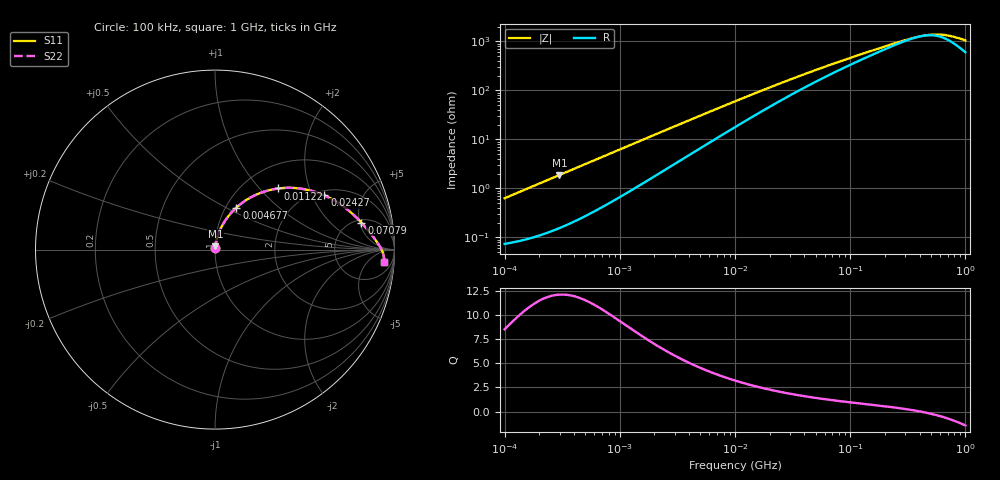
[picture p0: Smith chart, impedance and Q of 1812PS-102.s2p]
# MHz S MA R 50
!Freq  MagS11  AngS11  MagS21  AngS21  MagS12  AngS12  MagS22  AngS22
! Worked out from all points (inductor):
!   801 points, 100 kHz to 1 GHz, reference 50 ohm
!   read as one part in series: L = 999 nH near 104.7 kHz
!   highest Q = 12.1 at 298.5 kHz (marker M1), where L = 997 nH
!   self-resonance near 411 MHz
!   S11 on the Smith chart (normalised r, x): 100 kHz: 1.00, +0.01; 4.677 MHz: 1.12, +0.56; 11.22 MHz: 1.42, +1.27; 24.27 MHz: 2.20, +2.48; 70.79 MHz: 5.53, +5.32; 1 GHz: 13, -17
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0.1  0.006315 82.9  0.9992 -0.4  0.9992 -0.4  0.006315 82.9
0.2985383  0.01874 84.2  0.9983 -1.1  0.9983 -1.1  0.01874 84.2
0.4677351  0.02928 83.4  0.9971 -1.7  0.9971 -1.7  0.02928 83.4
1.083927  0.06716 79.9  0.9904 -3.8  0.9904 -3.8  0.06716 79.9
2.162719  0.1309 74.1  0.9724 -7.4  0.9724 -7.4  0.1309 74.1
3.273407  0.192 68.9  0.9479 -10.9  0.9479 -10.9  0.192 68.9
4.677351  0.2622 63.0  0.9116 -14.9  0.9116 -14.9  0.2622 63.0
6.76083  0.3513 55.7  0.853 -19.9  0.853 -19.9  0.3513 55.7
10  0.4582 46.8  0.7629 -25.9  0.7629 -25.9  0.4582 46.8
11.22018  0.4903 44.0  0.7314 -27.7  0.7314 -27.7  0.4903 44.0
16.2181  0.5885 35.2  0.6201 -33.2  0.6201 -33.2  0.5885 35.2
24.2661  0.68 26.4  0.494 -37.7  0.494 -37.7  0.68 26.4
33.49654  0.7381 20.4  0.4013 -39.8  0.4013 -39.8  0.7381 20.4
46.77351  0.7852 15.3  0.3189 -40.5  0.3189 -40.5  0.7852 15.3
70.79458  0.8294 10.4  0.2376 -39.2  0.2376 -39.2  0.8294 10.4
117.4898  0.8688 6.2  0.1655 -34.6  0.1655 -34.6  0.8688 6.2
216.2719  0.9027 2.8  0.1075 -23.8  0.1075 -23.8  0.9027 2.8
371.5352  0.9244 0.4  0.07595 -5.1  0.07595 -5.1  0.9244 0.4
518.8  0.9344 -1.0  0.06761 13.6  0.06761 13.6  0.9344 -1.0
602.5596  0.9381 -1.6  0.06777 23.2  0.06777 23.2  0.9381 -1.6
699.842  0.9411 -2.3  0.07081 32.6  0.07081 32.6  0.9411 -2.3
1000  0.9455 -4.2  0.09011 50.7  0.09011 50.7  0.9455 -4.2
